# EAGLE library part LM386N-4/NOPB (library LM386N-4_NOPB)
Linear IC - Audio amplifier Texas Instruments LM386N-4/NOPB 1-channel (mono) Class AB PDIP 8
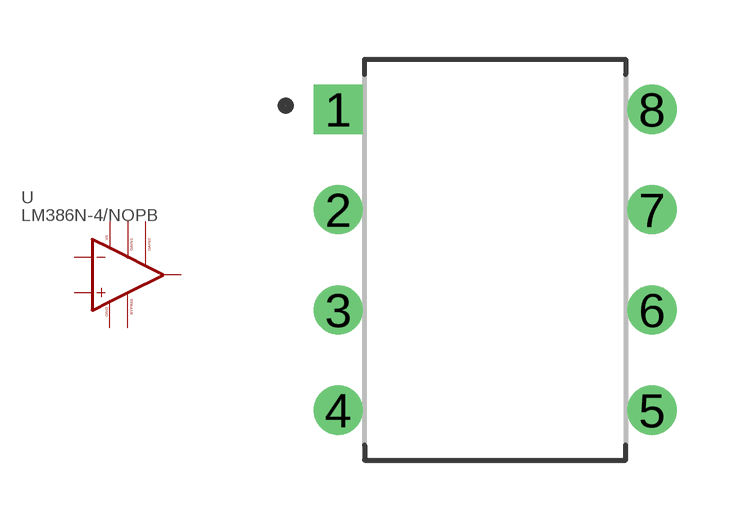
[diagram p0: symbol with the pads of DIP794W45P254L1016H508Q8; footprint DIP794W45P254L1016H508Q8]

Designator prefix U

## LM386N-4/NOPB (Availability: Unavailable; Description: Linear IC - Audio amplifier Texas Instruments LM386N-4/NOPB 1-channel _mono_ Class AB PDIP 8; MF: Texas Instruments; MP: LM386N-4/NOPB; Package: DIP-8 Texas Instruments; Price: None)  [DIP794W45P254L1016H508Q8]
1  GAIN1  pas
2  -INPUT  in
3  +INPUT  in
4  GND  pwr
5  VOUT  out
6  VS  pwr
7  BYPASS  out
8  GAIN2  pas

## Footprint DIP794W45P254L1016H508Q8 (pad centres in mm)
drill 0.74 pad 1.14 square: 1 -3.97,3.81
drill 0.74 pad 1.14: 2 -3.97,1.27; 3 -3.97,-1.27; 4 -3.97,-3.81; 5 3.97,-3.81; 6 3.97,-1.27; 7 3.97,1.27; 8 3.97,3.81

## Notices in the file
This work is licensed under a Creative Commons Attribution-ShareAlike 4.0 International License (CC BY-SA) with Design Exception 1.0
